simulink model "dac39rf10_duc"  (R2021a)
settings: Solver=FixedStepDiscrete  StartTime=0.0  StopTime=4136  RelTol=1e-3
StopFcn:
  | % Get interpolation factor from the L parameter on the DUC subsystem
  | duc = [gcs '/DUC']
  | Lstr = get_param(duc, 'L');
  | L = str2double(erase(Lstr, 'x'));
  | 
  | % Toss out 40*L output samples (40 input sample periods) for startup
  | N_in = size(dac_out,1)/L -40;
  | % Then assume input is bin-centered to the largest power of 2
  | N_in = 2^floor(log2(N_in));
  | % Multiply by L
  | N = N_in*L;
  | 
  | 
  | % Plot 2 channels
  | for ch = 0:1
  | 
  | 
  |     figure(ch+1);
  |     dac = dac_out(:,ch+1);
  |     dac_end = dac(end-N+1:end);
  |     f = [0:N/2];
  | 
  |     dac_fft = fft(dac_end/N*2);
  |     dac_fft = db( dac_fft(1:N/2+1) );
  |     dac_fft = max(dac_fft, -200*ones(N/2+1,1));
  | 
  |     plot(f, dac_fft);
  |     ylim([-150 3]);
  |     yticks([-200:10:0]);
  |     xlim([0 0.5]*N);
  |     xticks([0:0.5/8:0.5]*N);
  |     grid on;
  |     title(['DAC' num2str(ch) ' Output (' num2str(N) ' points)']);
  |     xlabel('Frequency Bin');
  |     ylabel('dBFS');
  | 
  | end
undefined symbols (not defined in the file): j, timearray
libraries: dspmlti4 x64, simulink x5
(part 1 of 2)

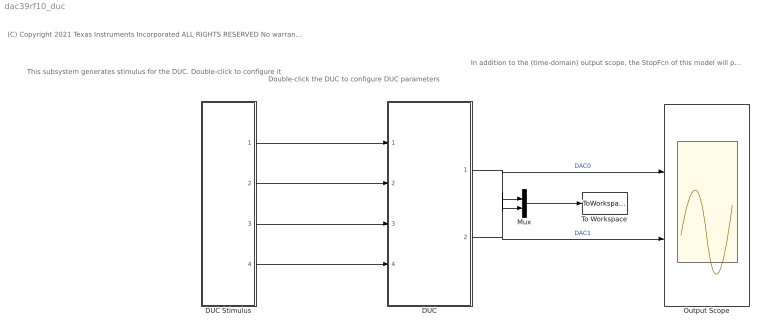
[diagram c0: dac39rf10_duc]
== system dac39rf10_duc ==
  note: Double-click the DUC to configure DUC parameters
  note: This subsystem generates stimulus for the DUC. Double-click to configure it
  note: In addition to the (time-domain) output scope, the StopFcn of this model will plot an FFT of the output
  note: (C) Copyright 2021 Texas Instruments Incorporated ALL RIGHTS RESERVED No warranty is expressed or implied
  DUC : Subsystem  mask{L=8x, DUC_FORMAT=off, FREQ0=0.25, FREQ1=0.25, FREQ2=0, FREQ3=0, PHASE0=0, PHASE1=0, PHASE2=0, PHASE3=0, DUC_GAIN0=-6dB, DUC_GAIN1=-6dB, DUC_GAIN2=0dB, DUC_GAIN3=0dB, DAC_SRC0_0=on, DAC_SRC0_1=on, DAC_SRC0_2=off, DAC_SRC0_3=off, DAC_SRC1_0=off, DAC_SRC1_1=on, DAC_SRC1_2=off, DAC_SRC1_3=off}
      mask prompts: L "Interpolation Factor"; DUC_FORMAT "Complex DUC Output (DUC_FORMAT=1)"; FREQ0 "Frequency (Ch 0) = 2^64 *"; FREQ1 "Frequency (Ch 1) = 2^64 *"; FREQ2 "Frequency (Ch 2) = 2^64 *"; FREQ3 "Frequency (Ch 3) = 2^64 *"; PHASE0 "Phase (Ch 0) = 2^16 *"; PHASE1 "Phase (Ch 1) = 2^16 *"; PHASE2 "Phase (Ch 2) = 2^16 *"; PHASE3 "Phase (Ch 3) = 2^16 *"; DAC_SRC0_0 "DUC0"; DAC_SRC0_1 "DUC1"; DAC_SRC0_2 "DUC2(real) / DUC0(imag)"; DAC_SRC0_3 "DUC3(real) / DUC1(imag)"; DAC_SRC1_0 "DUC0"; DAC_SRC1_1 "DUC1"; DAC_SRC1_2 "DUC2(real) / DUC0(imag)"; DAC_SRC1_3 "DUC3(real) / DUC1(imag)"
      mask help: DUC Model (DAC39RF10)
      mask init:
      | Lstr = get_param(gcb, 'L');
      | 
      | % Combine 4 frequency parameters into an array for the model to use
      | FREQ = [FREQ0 FREQ1 FREQ2 FREQ3];
      | 
      | PA_INIT = [PHASE0 PHASE1 PHASE2 PHASE3];
      | 
      | % Combine DAC_GAIN parameters
      | DUC_GAIN = [DUC_GAIN0 DUC_GAIN1 DUC_GAIN2 DUC_GAIN3];
      | 
      | % Convert 1->1, 2->0.5, 3->0.35
      | duc_gain = 2.^(1-DUC_GAIN);
      | 
      | % Combine DAC_SRC parameters into array for model
      | dac_src0 = [DAC_SRC0_0 DAC_SRC0_1 DAC_SRC0_2 DAC_SRC0_3];
      | dac_src1 = [DAC_SRC1_0 DAC_SRC1_1 DAC_SRC1_2 DAC_SRC1_3];
  DUC Stimulus : Subsystem  mask(Stimulus Block for DUC){N=4096, A0=0.99, F0=0.4, userData0=timearray, A1=0.99, F1=-0.4, userData1=, A2=0.99, F2=137/512, userData2=, A3=0.99, F3=137/512, userData3=}
      mask prompts: N "Sequence Length (N)"; A0 "Amplitude"; F0 "Frequency"; userData0 "User Data:"; A1 "Amplitude"; F1 "Frequency"; userData1 "User Data:"; A2 "Amplitude"; F2 "Frequency"; userData2 "User Data:"; A3 "Amplitude"; F3 "Frequency"; userData3 "User Data:"
      mask help: Specify Amplitudes and Frequencies for four IQ input channels. Sequency Length (N) should be a power of 2. The simulation stop time will be set to N+40 Amplitudes should be between 0.0 and 1.0 Frequencies units are [cycles per sample] (e.g. 1.0 = 2pi radians per sample) Frequencies outside the range of -0.5 to +0.5 will alias into that range. Frequencies will be rounded to make them coherent in N samples (length of input sequence) To provide custom stimulus, enter a variable name or MATLAB expression into the 'User Data' field. It will be evaluated in the base workspace, and should be a row or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
      mask init:
      | set_param(gcs, 'StopTime', num2str(N+40));
      | 
      | 
      | if( size(userData0,1) )
      |   duc0_input = evalin('base', userData0);
      | else
      |   duc0_input = A0*exp(j*round(F0*N)/N*2*pi*[0:N-1]) + (rand(1,N)-0.5)*2^-15;    
      | end
      | 
      | if( size(userData1,1) )
      |   duc1_input = evalin('base', userData1);
      | else
      |   duc1_input = A1*exp(j*round(F1*N)/N*2*pi*[0:N-1]) + (rand(1,N)-0.5)*2^-15;    
      | end
      | 
      | if( size(userData2,1) )
      |   duc2_input = evalin('base', userData2);
      | else
      |   duc2_input = A2*exp(j*round(F2*N)/N*2*pi*[0:N-1]) + (rand(1,N)-0.5)*2^-15;    
      | end
      | 
      | if( size(userData3,1) )
      |   duc3_input = evalin('base', userData3);
      | else
      |   duc3_input = A3*exp(j*round(F3*N)/N*2*pi*[0:N-1]) + (rand(1,N)-0.5)*2^-15;    
      | end
  Mux : Mux  Inputs=2
  Output Scope : Scope  NumInputPorts=2
  To Workspace : ToWorkspace  VariableName=dac_out  SampleTime=-1
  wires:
  DUC/1(Out1) -> Mux/1, Output Scope/1  "DAC0"
  DUC/2(Out2) -> Mux/2, Output Scope/2  "DAC1"
  Mux/1 -> To Workspace/1
  DUC Stimulus/1(Ch0) -> DUC/1(Ch0)
  DUC Stimulus/2(Ch1) -> DUC/2(Ch1)
  DUC Stimulus/3(Ch2) -> DUC/3(Ch2)
  DUC Stimulus/4(Ch3) -> DUC/4(Ch3)

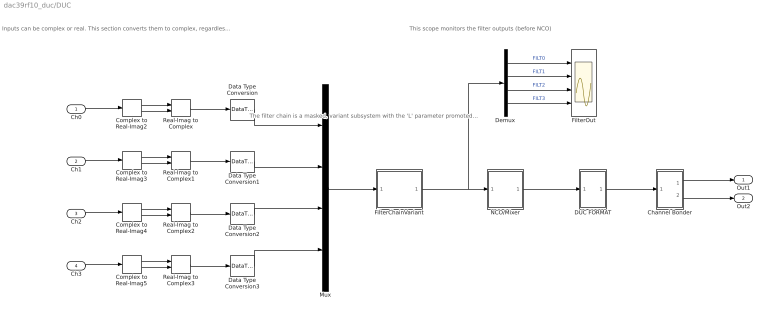
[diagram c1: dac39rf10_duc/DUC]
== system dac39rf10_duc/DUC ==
  note: This scope monitors the filter outputs (before NCO)
  note: The filter chain is a masked, variant subsystem with the 'L' parameter promoted up to the DUC mask
  note: Inputs can be complex or real. This section converts them to complex, regardless of what format they are initially in.
  Ch0 : Inport
  Ch1 : Inport  Port=2
  Ch2 : Inport  Port=3
  Ch3 : Inport  Port=4
  Channel Bonder : Subsystem
  Complex to Real-Imag{2..5} (4 alike) : ComplexToRealImag
  DUC FORMAT : Subsystem
  Data Type Conversion{,1..3} (4 alike) : DataTypeConversion  OutDataTypeStr=fixdt(1,16,15)  RndMeth=Round
  Demux : Demux
  FilterChainVariant : Subsystem  Variant=on  VariantControlMode=label  VariantControl=Variant1  LabelModeActiveChoice=var8x  mask{L=8x}
      mask prompts: L "Interpolation Factor"
      mask init:
      | simulationStatus =  get_param(bdroot,'SimulationStatus');
      | 
      | % The active variant can only be modified at edit-time or very early during
      | % the simulink compile stage. 
      | 
      |    % The L parameter is just an index into a list of strings. This gets the
      |    % string
      |    Lstr = get_param(gcb, 'L');  
      |    set_param(gcb, 'OverrideUsingVariant', ['var', Lstr]);
  FilterOut : Scope  NumInputPorts=4
  Mux : Mux
  NCO/Mixer : Subsystem
  Real-Imag to Complex{,1..3} (4 alike) : RealImagToComplex
  Out1 : Outport  VectorParamsAs1DForOutWhenUnconnected=off
  Out2 : Outport  Port=2  VectorParamsAs1DForOutWhenUnconnected=off
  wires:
  Demux/2 -> FilterOut/2  "FILT1"
  Demux/1 -> FilterOut/1  "FILT0"
  Mux/1 -> FilterChainVariant/1("In1 ")
  Complex to Real-Imag2/1 -> Real-Imag to Complex/1
  Complex to Real-Imag2/2 -> Real-Imag to Complex/2
  Complex to Real-Imag3/2 -> Real-Imag to Complex1/2
  Complex to Real-Imag3/1 -> Real-Imag to Complex1/1
  Complex to Real-Imag4/1 -> Real-Imag to Complex2/1
  Complex to Real-Imag4/2 -> Real-Imag to Complex2/2
  Complex to Real-Imag5/2 -> Real-Imag to Complex3/2
  Complex to Real-Imag5/1 -> Real-Imag to Complex3/1
  Ch0/1 -> Complex to Real-Imag2/1
  Ch1/1 -> Complex to Real-Imag3/1
  Ch2/1 -> Complex to Real-Imag4/1
  Ch3/1 -> Complex to Real-Imag5/1
  Real-Imag to Complex/1 -> Data Type Conversion/1
  Real-Imag to Complex1/1 -> Data Type Conversion1/1
  Real-Imag to Complex2/1 -> Data Type Conversion2/1
  Real-Imag to Complex3/1 -> Data Type Conversion3/1
  FilterChainVariant/1(" Out1") -> Demux/1, NCO/Mixer/1(In1)
  NCO/Mixer/1(Out1) -> DUC FORMAT/1(In1)
  DUC FORMAT/1(Out1) -> Channel Bonder/1(In1)
  Channel Bonder/1(Out1) -> Out1/1
  Channel Bonder/2(Out2) -> Out2/1
  Demux/3 -> FilterOut/3  "FILT2"
  Demux/4 -> FilterOut/4  "FILT3"
  Data Type Conversion/1 -> Mux/1
  Data Type Conversion1/1 -> Mux/2
  Data Type Conversion2/1 -> Mux/3
  Data Type Conversion3/1 -> Mux/4

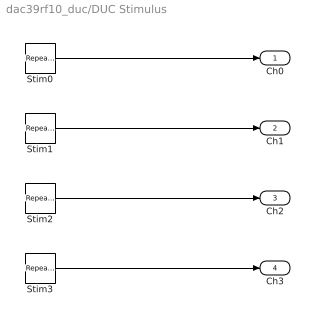
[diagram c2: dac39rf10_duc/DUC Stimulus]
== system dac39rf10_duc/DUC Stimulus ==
  Stim0 : simulink/Sources/Repeating Sequence Stair  OutValues=duc0_input  tsamp=1  OutMin=[]  OutMax=[]  OutDataTypeStr=double  OutputDataTypeScalingMode=double  OutDataType=fixdt(0,8)  ConRadixGroup=Best Precision: Vector-wise  OutScaling=2^-12
  Stim1 : simulink/Sources/Repeating Sequence Stair  OutValues=duc1_input  tsamp=1  OutMin=[]  OutMax=[]  OutDataTypeStr=double  OutputDataTypeScalingMode=double  OutDataType=fixdt(0,8)  ConRadixGroup=Best Precision: Vector-wise  OutScaling=2^-12
  Stim2 : simulink/Sources/Repeating Sequence Stair  OutValues=duc2_input  tsamp=1  OutMin=[]  OutMax=[]  OutDataTypeStr=double  OutputDataTypeScalingMode=double  OutDataType=fixdt(0,8)  ConRadixGroup=Best Precision: Vector-wise  OutScaling=2^-12
  Stim3 : simulink/Sources/Repeating Sequence Stair  OutValues=duc3_input  tsamp=1  OutMin=[]  OutMax=[]  OutDataTypeStr=double  OutputDataTypeScalingMode=double  OutDataType=fixdt(0,8)  ConRadixGroup=Best Precision: Vector-wise  OutScaling=2^-12
  Ch0 : Outport  VectorParamsAs1DForOutWhenUnconnected=off
  Ch1 : Outport  Port=2  VectorParamsAs1DForOutWhenUnconnected=off
  Ch2 : Outport  Port=3  VectorParamsAs1DForOutWhenUnconnected=off
  Ch3 : Outport  Port=4  VectorParamsAs1DForOutWhenUnconnected=off
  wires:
  Stim1/1 -> Ch1/1
  Stim2/1 -> Ch2/1
  Stim3/1 -> Ch3/1
  Stim0/1 -> Ch0/1

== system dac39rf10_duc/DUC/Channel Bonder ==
  note: DUC_GAIN is done with elementwise multiplication
  note: DAC_SRC is done with matrix multiplication (1x4 * 4x1 = 1x1)
  In1 : Inport  PortDimensions=4
  DAC_SRC0 : Gain  Gain=dac_src0  Multiplication=Matrix(K*u)  OutDataTypeStr=fixdt(1,16,15)  RndMeth=Nearest
  DAC_SRC1 : Gain  Gain=dac_src1  Multiplication=Matrix(K*u)  OutDataTypeStr=fixdt(1,16,15)  RndMeth=Nearest
  DUC_GAIN : Gain  Gain=duc_gain  OutDataTypeStr=fixdt(1,18,17)
  Out1 : Outport  VectorParamsAs1DForOutWhenUnconnected=off
  Out2 : Outport  Port=2  VectorParamsAs1DForOutWhenUnconnected=off
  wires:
  DAC_SRC0/1 -> Out1/1
  DUC_GAIN/1 -> DAC_SRC1/1, DAC_SRC0/1
  DAC_SRC1/1 -> Out2/1
  In1/1 -> DUC_GAIN/1

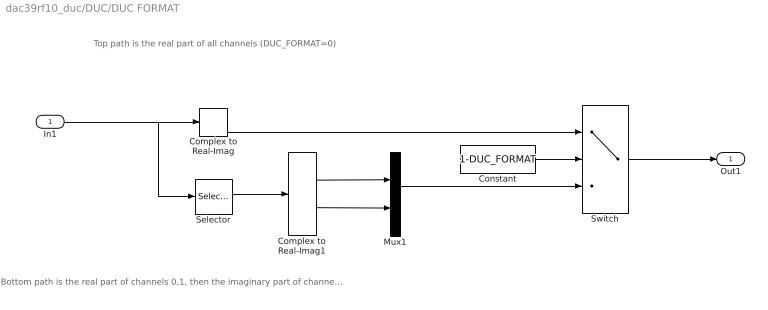
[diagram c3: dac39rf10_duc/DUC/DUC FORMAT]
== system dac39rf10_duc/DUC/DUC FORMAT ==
  note: Bottom path is the real part of channels 0,1, then the imaginary part of channels 0 and 1 (DUC_FORMAT=1)
  note: Top path is the real part of all channels (DUC_FORMAT=0)
  In1 : Inport  PortDimensions=4
  Complex to Real-Imag : ComplexToRealImag  Output=Real
  Complex to Real-Imag1 : ComplexToRealImag
  Constant : Constant  Value=1-DUC_FORMAT
  Mux1 : Mux  Inputs=2
  Selector : Selector  InputPortWidth=4  IndexOptions=Index vector (dialog)  Indices=[1 2]  OutputSizes=1
  Switch : Switch  Criteria=u2 > Threshold
  Out1 : Outport  PortDimensions=4  VectorParamsAs1DForOutWhenUnconnected=off
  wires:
  Mux1/1 -> Switch/3
  Complex to Real-Imag/1 -> Switch/1
  Complex to Real-Imag1/1 -> Mux1/1
  Selector/1 -> Complex to Real-Imag1/1
  In1/1 -> Selector/1, Complex to Real-Imag/1
  Switch/1 -> Out1/1
  Complex to Real-Imag1/2 -> Mux1/2
  Constant/1 -> Switch/2

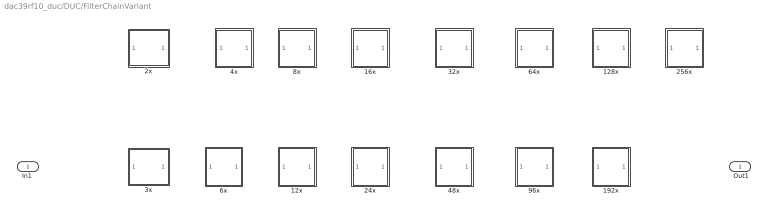
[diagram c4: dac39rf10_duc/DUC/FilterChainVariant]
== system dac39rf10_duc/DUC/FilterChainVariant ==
  "In1 " : Inport
  128x : Subsystem  VariantControl=var128x
  12x : Subsystem  VariantControl=var12x
  16x : Subsystem  VariantControl=var16x
  192x : Subsystem  VariantControl=var192x
  24x : Subsystem  VariantControl=var24x
  256x : Subsystem  VariantControl=var256x
  2x : Subsystem  VariantControl=var2x
  32x : Subsystem  VariantControl=var32x
  3x : Subsystem  VariantControl=var3x
  48x : Subsystem  VariantControl=var48x
  4x : Subsystem  VariantControl=var4x
  64x : Subsystem  VariantControl=var64x
  6x : Subsystem  VariantControl=var6x
  8x : Subsystem  VariantControl=var8x
  96x : Subsystem  VariantControl=var96x
  " Out1" : Outport  VectorParamsAs1DForOutWhenUnconnected=off

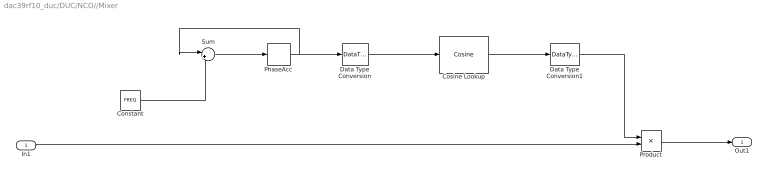
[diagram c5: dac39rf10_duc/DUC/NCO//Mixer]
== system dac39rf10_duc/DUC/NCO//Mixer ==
  In1 : Inport
  Constant : Constant  Value=FREQ  OutDataTypeStr=fixdt(0,64,64)
  Cosine Lookup : simulink/Lookup Tables/Cosine  Formula=exp(j*2*pi*u)  NumDataPoints=(2^18)+1  OutputWordLength=20  InternalRulePriority=Precision
  Data Type Conversion : DataTypeConversion  OutDataTypeStr=fixdt(0,18,18)
  Data Type Conversion1 : DataTypeConversion  OutDataTypeStr=fixdt(1,17,15)  RndMeth=Nearest
  PhaseAcc : Delay  DelayLength=1  InitialCondition=PA_INIT
  Product : Product  OutDataTypeStr=fixdt(1,16,15)  RndMeth=Nearest  SaturateOnIntegerOverflow=on
  Sum : Sum  Inputs=|++  OutDataTypeStr=fixdt(0,64,64)
  Out1 : Outport  VectorParamsAs1DForOutWhenUnconnected=off
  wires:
  PhaseAcc/1 -> Sum/1, Data Type Conversion/1
  Product/1 -> Out1/1
  In1/1 -> Product/2
  Cosine Lookup/1 -> Data Type Conversion1/1
  Data Type Conversion1/1 -> Product/1
  Sum/1 -> PhaseAcc/1
  Data Type Conversion/1 -> Cosine Lookup/1
  Constant/1 -> Sum/2

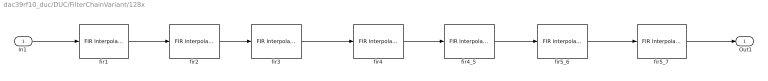
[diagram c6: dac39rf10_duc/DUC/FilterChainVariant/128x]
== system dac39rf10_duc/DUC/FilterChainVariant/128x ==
  "In1 " : Inport
  fir1 : dspmlti4/FIR Interpolation  FilterSource=Dialog parameters  h=[6 0 -19 0 47 0 -100 0 192 0 -342 0 572 0 -914 0 1409 0 -2119 0 3152 0 -4729 0 7420 0 -13334 0 41527 65536 41527 0 -13334 0 7420 0 -4729 0 3152 0 -2119 0 1409 0 -914 0 572 0 -342 0 192 0 -100 0 47 0 -19 0 6 ]*2^-16  L=2  FilterObject=FINTERP  framing=Enforce single-rate processing  outputBufInitCond=0  roundingMode=Round  overflowMode=on  firstCoeffMode=Binary point scaling  firstCoeffWordLength=18  firstCoeffFracLength=16  firstCoeffDataTypeStr=fixdt(1,18,16)  firstCoeffMin=[]  firstCoeffMax=[]  firstCoeffLastDataTypeStr=fixdt(1,18,16)  outputMode=Binary point scaling  outputWordLength=18  outputFracLength=17  outputDataTypeStr=fixdt(1,18,17)  outputMin=[]  outputMax=[]  outputLastDataTypeStr=fixdt(1,18,17)
  fir2 : dspmlti4/FIR Interpolation  FilterSource=Dialog parameters  h=[-12 0 84 0 -336 0 1006 0 -2691 0 10141 16384 10141 0 -2691 0 1006 0 -336 0 84 0 -12 ]*2^-14  L=2  FilterObject=FINTERP  framing=Enforce single-rate processing  outputBufInitCond=0  roundingMode=Round  overflowMode=on  firstCoeffMode=Binary point scaling  firstCoeffWordLength=16  firstCoeffFracLength=14  firstCoeffDataTypeStr=fixdt(1,16,14)  firstCoeffMin=[]  firstCoeffMax=[]  firstCoeffLastDataTypeStr=fixdt(1,16,14)  outputMode=Binary point scaling  outputWordLength=18  outputFracLength=17  outputDataTypeStr=fixdt(1,18,17)  outputMin=[]  outputMax=[]  outputLastDataTypeStr=fixdt(1,18,17)
  fir3 : dspmlti4/FIR Interpolation  FilterSource=Dialog parameters  h=[29 0 -214 0 1209 2048 1209 0 -214 0 29 ]*2^-11  L=2  FilterObject=FINTERP  framing=Enforce single-rate processing  outputBufInitCond=0  roundingMode=Round  overflowMode=on  firstCoeffMode=Binary point scaling  firstCoeffWordLength=13  firstCoeffFracLength=11  firstCoeffDataTypeStr=fixdt(1,13,11)  firstCoeffMin=[]  firstCoeffMax=[]  firstCoeffLastDataTypeStr=fixdt(1,13,11)  outputMode=Binary point scaling  outputWordLength=17  outputFracLength=16  outputDataTypeStr=fixdt(1,17,16)  outputMin=[]  outputMax=[]  outputLastDataTypeStr=fixdt(1,17,16)
  fir4 : dspmlti4/FIR Interpolation  FilterSource=Dialog parameters  h=[3 0 -25 0 150 256 150 0 -25 0 3 ]*2^-8  L=2  FilterObject=FINTERP  framing=Enforce single-rate processing  outputBufInitCond=0  roundingMode=Round  overflowMode=on  firstCoeffMode=Binary point scaling  firstCoeffWordLength=10  firstCoeffFracLength=8  firstCoeffDataTypeStr=fixdt(1,10,8)  firstCoeffMin=[]  firstCoeffMax=[]  firstCoeffLastDataTypeStr=fixdt(1,10,8)  outputMode=Binary point scaling  outputWordLength=17  outputFracLength=16  outputDataTypeStr=fixdt(1,17,16)  outputMin=[]  outputMax=[]  outputLastDataTypeStr=fixdt(1,17,16)
  fir4_5 : dspmlti4/FIR Interpolation  FilterSource=Dialog parameters  h=[3 0 -25 0 150 256 150 0 -25 0 3 ]*2^-8  L=2  FilterObject=FINTERP  framing=Enforce single-rate processing  outputBufInitCond=0  roundingMode=Round  overflowMode=on  firstCoeffMode=Binary point scaling  firstCoeffWordLength=10  firstCoeffFracLength=8  firstCoeffDataTypeStr=fixdt(1,10,8)  firstCoeffMin=[]  firstCoeffMax=[]  firstCoeffLastDataTypeStr=fixdt(1,10,8)  outputMode=Binary point scaling  outputWordLength=17  outputFracLength=16  outputDataTypeStr=fixdt(1,17,16)  outputMin=[]  outputMax=[]  outputLastDataTypeStr=fixdt(1,17,16)
  fir5_6 : dspmlti4/FIR Interpolation  FilterSource=Dialog parameters  h=[-1 0 9 16 9 0 -1]*2^-4  L=2  FilterObject=FINTERP  framing=Enforce single-rate processing  outputBufInitCond=0  roundingMode=Round  overflowMode=on  firstCoeffMode=Binary point scaling  firstCoeffWordLength=6  firstCoeffFracLength=4  firstCoeffDataTypeStr=fixdt(1,6,4)  firstCoeffMin=[]  firstCoeffMax=[]  firstCoeffLastDataTypeStr=fixdt(1,6,4)  outputMode=Binary point scaling  outputWordLength=16  outputFracLength=15  outputDataTypeStr=fixdt(1,16,15)  outputMin=[]  outputMax=[]  outputLastDataTypeStr=fixdt(1,16,15)
  fir5_7 : dspmlti4/FIR Interpolation  FilterSource=Dialog parameters  h=[-1 0 9 16 9 0 -1]*2^-4  L=2  FilterObject=FINTERP  framing=Enforce single-rate processing  outputBufInitCond=0  roundingMode=Round  overflowMode=on  firstCoeffMode=Binary point scaling  firstCoeffWordLength=6  firstCoeffFracLength=4  firstCoeffDataTypeStr=fixdt(1,6,4)  firstCoeffMin=[]  firstCoeffMax=[]  firstCoeffLastDataTypeStr=fixdt(1,6,4)  outputMode=Binary point scaling  outputWordLength=16  outputFracLength=15  outputDataTypeStr=fixdt(1,16,15)  outputMin=[]  outputMax=[]  outputLastDataTypeStr=fixdt(1,16,15)
  " Out1" : Outport  VectorParamsAs1DForOutWhenUnconnected=off
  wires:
  fir5_7/1 -> " Out1"/1
  fir4/1 -> fir4_5/1
  fir3/1 -> fir4/1
  fir2/1 -> fir3/1
  fir1/1 -> fir2/1
  "In1 "/1 -> fir1/1
  fir5_6/1 -> fir5_7/1
  fir4_5/1 -> fir5_6/1

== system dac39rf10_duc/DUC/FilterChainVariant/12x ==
  "In1 " : Inport
  fir2 : dspmlti4/FIR Interpolation  FilterSource=Dialog parameters  h=[-12 0 84 0 -336 0 1006 0 -2691 0 10141 16384 10141 0 -2691 0 1006 0 -336 0 84 0 -12 ]*2^-14  L=2  FilterObject=FINTERP  framing=Enforce single-rate processing  outputBufInitCond=0  roundingMode=Round  overflowMode=on  firstCoeffMode=Binary point scaling  firstCoeffWordLength=16  firstCoeffFracLength=14  firstCoeffDataTypeStr=fixdt(1,16,14)  firstCoeffMin=[]  firstCoeffMax=[]  firstCoeffLastDataTypeStr=fixdt(1,16,14)  outputMode=Binary point scaling  outputWordLength=18  outputFracLength=17  outputDataTypeStr=fixdt(1,18,17)  outputMin=[]  outputMax=[]  outputLastDataTypeStr=fixdt(1,18,17)
  fir3 : dspmlti4/FIR Interpolation  FilterSource=Dialog parameters  h=[29 0 -214 0 1209 2048 1209 0 -214 0 29 ]*2^-11  L=2  FilterObject=FINTERP  framing=Enforce single-rate processing  outputBufInitCond=0  roundingMode=Round  overflowMode=on  firstCoeffMode=Binary point scaling  firstCoeffWordLength=13  firstCoeffFracLength=11  firstCoeffDataTypeStr=fixdt(1,13,11)  firstCoeffMin=[]  firstCoeffMax=[]  firstCoeffLastDataTypeStr=fixdt(1,13,11)  outputMode=Binary point scaling  outputWordLength=16  outputFracLength=15  outputDataTypeStr=fixdt(1,16,15)  outputMin=[]  outputMax=[]  outputLastDataTypeStr=fixdt(1,16,15)
  fir3x : dspmlti4/FIR Interpolation  FilterSource=Dialog parameters  h=[-38 -38 0 83 117 0 -214 -281 0 464 584 0 -900 -1102 0 1612 1929 0 -2713 -3190 0 4346 5040 0 -6699 -7684 0 10023 11408 0 -14701 -16661 0 21389 24260 0 -31417 -35960 0 48101 56540 0 -82781 -105224 0 215190 432780 524288 432780 215190 0 -105224 -82781 0 56540 48101 0 -35960 -31417 0 24260 21389 0 -16661 -14701 0 11408 10023 0 -7684 -6699 0 5040 4346 0 -3190 -2713 0 1929 1612 0 -1102 -900 0 584 464 0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  L=3  FilterObject=FINTERP  framing=Enforce single-rate processing  outputBufInitCond=0  roundingMode=Round  overflowMode=on  firstCoeffMode=Binary point scaling  firstCoeffWordLength=21  firstCoeffFracLength=19  firstCoeffDataTypeStr=fixdt(1,21,19)  firstCoeffMin=[]  firstCoeffMax=[]  firstCoeffLastDataTypeStr=fixdt(1,21,19)  outputMode=Binary point scaling  outputWordLength=18  outputFracLength=17  outputDataTypeStr=fixdt(1,18,17)  outputMin=[]  outputMax=[]  outputLastDataTypeStr=fixdt(1,18,17)
  " Out1" : Outport  VectorParamsAs1DForOutWhenUnconnected=off
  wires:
  fir3/1 -> " Out1"/1
  "In1 "/1 -> fir3x/1
  fir3x/1 -> fir2/1
  fir2/1 -> fir3/1

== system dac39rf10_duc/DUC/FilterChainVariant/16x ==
  "In1 " : Inport
  fir1 : dspmlti4/FIR Interpolation  FilterSource=Dialog parameters  h=[6 0 -19 0 47 0 -100 0 192 0 -342 0 572 0 -914 0 1409 0 -2119 0 3152 0 -4729 0 7420 0 -13334 0 41527 65536 41527 0 -13334 0 7420 0 -4729 0 3152 0 -2119 0 1409 0 -914 0 572 0 -342 0 192 0 -100 0 47 0 -19 0 6 ]*2^-16  L=2  FilterObject=FINTERP  framing=Enforce single-rate processing  outputBufInitCond=0  roundingMode=Round  overflowMode=on  firstCoeffMode=Binary point scaling  firstCoeffWordLength=18  firstCoeffFracLength=16  firstCoeffDataTypeStr=fixdt(1,18,16)  firstCoeffMin=[]  firstCoeffMax=[]  firstCoeffLastDataTypeStr=fixdt(1,18,16)  outputMode=Binary point scaling  outputWordLength=18  outputFracLength=17  outputDataTypeStr=fixdt(1,18,17)  outputMin=[]  outputMax=[]  outputLastDataTypeStr=fixdt(1,18,17)
  fir2 : dspmlti4/FIR Interpolation  FilterSource=Dialog parameters  h=[-12 0 84 0 -336 0 1006 0 -2691 0 10141 16384 10141 0 -2691 0 1006 0 -336 0 84 0 -12 ]*2^-14  L=2  FilterObject=FINTERP  framing=Enforce single-rate processing  outputBufInitCond=0  roundingMode=Round  overflowMode=on  firstCoeffMode=Binary point scaling  firstCoeffWordLength=16  firstCoeffFracLength=14  firstCoeffDataTypeStr=fixdt(1,16,14)  firstCoeffMin=[]  firstCoeffMax=[]  firstCoeffLastDataTypeStr=fixdt(1,16,14)  outputMode=Binary point scaling  outputWordLength=18  outputFracLength=17  outputDataTypeStr=fixdt(1,18,17)  outputMin=[]  outputMax=[]  outputLastDataTypeStr=fixdt(1,18,17)
  fir3 : dspmlti4/FIR Interpolation  FilterSource=Dialog parameters  h=[29 0 -214 0 1209 2048 1209 0 -214 0 29 ]*2^-11  L=2  FilterObject=FINTERP  framing=Enforce single-rate processing  outputBufInitCond=0  roundingMode=Round  overflowMode=on  firstCoeffMode=Binary point scaling  firstCoeffWordLength=13  firstCoeffFracLength=11  firstCoeffDataTypeStr=fixdt(1,13,11)  firstCoeffMin=[]  firstCoeffMax=[]  firstCoeffLastDataTypeStr=fixdt(1,13,11)  outputMode=Binary point scaling  outputWordLength=17  outputFracLength=16  outputDataTypeStr=fixdt(1,17,16)  outputMin=[]  outputMax=[]  outputLastDataTypeStr=fixdt(1,17,16)
  fir4 : dspmlti4/FIR Interpolation  FilterSource=Dialog parameters  h=[3 0 -25 0 150 256 150 0 -25 0 3 ]*2^-8  L=2  FilterObject=FINTERP  framing=Enforce single-rate processing  outputBufInitCond=0  roundingMode=Round  overflowMode=on  firstCoeffMode=Binary point scaling  firstCoeffWordLength=10  firstCoeffFracLength=8  firstCoeffDataTypeStr=fixdt(1,10,8)  firstCoeffMin=[]  firstCoeffMax=[]  firstCoeffLastDataTypeStr=fixdt(1,10,8)  outputMode=Binary point scaling  outputWordLength=16  outputFracLength=15  outputDataTypeStr=fixdt(1,16,15)  outputMin=[]  outputMax=[]  outputLastDataTypeStr=fixdt(1,16,15)
  " Out1" : Outport  VectorParamsAs1DForOutWhenUnconnected=off
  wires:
  "In1 "/1 -> fir1/1
  fir1/1 -> fir2/1
  fir2/1 -> fir3/1
  fir3/1 -> fir4/1
  fir4/1 -> " Out1"/1

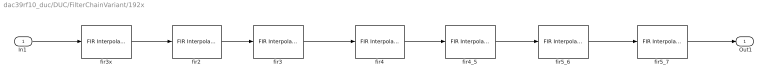
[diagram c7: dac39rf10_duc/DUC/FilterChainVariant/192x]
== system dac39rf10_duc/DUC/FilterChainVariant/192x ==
  "In1 " : Inport
  fir2 : dspmlti4/FIR Interpolation  FilterSource=Dialog parameters  h=[-12 0 84 0 -336 0 1006 0 -2691 0 10141 16384 10141 0 -2691 0 1006 0 -336 0 84 0 -12 ]*2^-14  L=2  FilterObject=FINTERP  framing=Enforce single-rate processing  outputBufInitCond=0  roundingMode=Round  overflowMode=on  firstCoeffMode=Binary point scaling  firstCoeffWordLength=16  firstCoeffFracLength=14  firstCoeffDataTypeStr=fixdt(1,16,14)  firstCoeffMin=[]  firstCoeffMax=[]  firstCoeffLastDataTypeStr=fixdt(1,16,14)  outputMode=Binary point scaling  outputWordLength=18  outputFracLength=17  outputDataTypeStr=fixdt(1,18,17)  outputMin=[]  outputMax=[]  outputLastDataTypeStr=fixdt(1,18,17)
  fir3 : dspmlti4/FIR Interpolation  FilterSource=Dialog parameters  h=[29 0 -214 0 1209 2048 1209 0 -214 0 29 ]*2^-11  L=2  FilterObject=FINTERP  framing=Enforce single-rate processing  outputBufInitCond=0  roundingMode=Round  overflowMode=on  firstCoeffMode=Binary point scaling  firstCoeffWordLength=13  firstCoeffFracLength=11  firstCoeffDataTypeStr=fixdt(1,13,11)  firstCoeffMin=[]  firstCoeffMax=[]  firstCoeffLastDataTypeStr=fixdt(1,13,11)  outputMode=Binary point scaling  outputWordLength=17  outputFracLength=16  outputDataTypeStr=fixdt(1,17,16)  outputMin=[]  outputMax=[]  outputLastDataTypeStr=fixdt(1,17,16)
  fir3x : dspmlti4/FIR Interpolation  FilterSource=Dialog parameters  h=[-38 -38 0 83 117 0 -214 -281 0 464 584 0 -900 -1102 0 1612 1929 0 -2713 -3190 0 4346 5040 0 -6699 -7684 0 10023 11408 0 -14701 -16661 0 21389 24260 0 -31417 -35960 0 48101 56540 0 -82781 -105224 0 215190 432780 524288 432780 215190 0 -105224 -82781 0 56540 48101 0 -35960 -31417 0 24260 21389 0 -16661 -14701 0 11408 10023 0 -7684 -6699 0 5040 4346 0 -3190 -2713 0 1929 1612 0 -1102 -900 0 584 464 0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  L=3  FilterObject=FINTERP  framing=Enforce single-rate processing  outputBufInitCond=0  roundingMode=Round  overflowMode=on  firstCoeffMode=Binary point scaling  firstCoeffWordLength=21  firstCoeffFracLength=19  firstCoeffDataTypeStr=fixdt(1,21,19)  firstCoeffMin=[]  firstCoeffMax=[]  firstCoeffLastDataTypeStr=fixdt(1,21,19)  outputMode=Binary point scaling  outputWordLength=18  outputFracLength=17  outputDataTypeStr=fixdt(1,18,17)  outputMin=[]  outputMax=[]  outputLastDataTypeStr=fixdt(1,18,17)
  fir4 : dspmlti4/FIR Interpolation  FilterSource=Dialog parameters  h=[3 0 -25 0 150 256 150 0 -25 0 3 ]*2^-8  L=2  FilterObject=FINTERP  framing=Enforce single-rate processing  outputBufInitCond=0  roundingMode=Round  overflowMode=on  firstCoeffMode=Binary point scaling  firstCoeffWordLength=10  firstCoeffFracLength=8  firstCoeffDataTypeStr=fixdt(1,10,8)  firstCoeffMin=[]  firstCoeffMax=[]  firstCoeffLastDataTypeStr=fixdt(1,10,8)  outputMode=Binary point scaling  outputWordLength=17  outputFracLength=16  outputDataTypeStr=fixdt(1,17,16)  outputMin=[]  outputMax=[]  outputLastDataTypeStr=fixdt(1,17,16)
  fir4_5 : dspmlti4/FIR Interpolation  FilterSource=Dialog parameters  h=[3 0 -25 0 150 256 150 0 -25 0 3 ]*2^-8  L=2  FilterObject=FINTERP  framing=Enforce single-rate processing  outputBufInitCond=0  roundingMode=Round  overflowMode=on  firstCoeffMode=Binary point scaling  firstCoeffWordLength=10  firstCoeffFracLength=8  firstCoeffDataTypeStr=fixdt(1,10,8)  firstCoeffMin=[]  firstCoeffMax=[]  firstCoeffLastDataTypeStr=fixdt(1,10,8)  outputMode=Binary point scaling  outputWordLength=17  outputFracLength=16  outputDataTypeStr=fixdt(1,17,16)  outputMin=[]  outputMax=[]  outputLastDataTypeStr=fixdt(1,17,16)
  fir5_6 : dspmlti4/FIR Interpolation  FilterSource=Dialog parameters  h=[-1 0 9 16 9 0 -1]*2^-4  L=2  FilterObject=FINTERP  framing=Enforce single-rate processing  outputBufInitCond=0  roundingMode=Round  overflowMode=on  firstCoeffMode=Binary point scaling  firstCoeffWordLength=6  firstCoeffFracLength=4  firstCoeffDataTypeStr=fixdt(1,6,4)  firstCoeffMin=[]  firstCoeffMax=[]  firstCoeffLastDataTypeStr=fixdt(1,6,4)  outputMode=Binary point scaling  outputWordLength=16  outputFracLength=15  outputDataTypeStr=fixdt(1,16,15)  outputMin=[]  outputMax=[]  outputLastDataTypeStr=fixdt(1,16,15)
  fir5_7 : dspmlti4/FIR Interpolation  FilterSource=Dialog parameters  h=[-1 0 9 16 9 0 -1]*2^-4  L=2  FilterObject=FINTERP  framing=Enforce single-rate processing  outputBufInitCond=0  roundingMode=Round  overflowMode=on  firstCoeffMode=Binary point scaling  firstCoeffWordLength=6  firstCoeffFracLength=4  firstCoeffDataTypeStr=fixdt(1,6,4)  firstCoeffMin=[]  firstCoeffMax=[]  firstCoeffLastDataTypeStr=fixdt(1,6,4)  outputMode=Binary point scaling  outputWordLength=16  outputFracLength=15  outputDataTypeStr=fixdt(1,16,15)  outputMin=[]  outputMax=[]  outputLastDataTypeStr=fixdt(1,16,15)
  " Out1" : Outport  VectorParamsAs1DForOutWhenUnconnected=off
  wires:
  fir4_5/1 -> fir5_6/1
  fir5_6/1 -> fir5_7/1
  "In1 "/1 -> fir3x/1
  fir3x/1 -> fir2/1
  fir2/1 -> fir3/1
  fir3/1 -> fir4/1
  fir4/1 -> fir4_5/1
  fir5_7/1 -> " Out1"/1

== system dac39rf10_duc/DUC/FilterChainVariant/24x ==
  "In1 " : Inport
  fir2 : dspmlti4/FIR Interpolation  FilterSource=Dialog parameters  h=[-12 0 84 0 -336 0 1006 0 -2691 0 10141 16384 10141 0 -2691 0 1006 0 -336 0 84 0 -12 ]*2^-14  L=2  FilterObject=FINTERP  framing=Enforce single-rate processing  outputBufInitCond=0  roundingMode=Round  overflowMode=on  firstCoeffMode=Binary point scaling  firstCoeffWordLength=16  firstCoeffFracLength=14  firstCoeffDataTypeStr=fixdt(1,16,14)  firstCoeffMin=[]  firstCoeffMax=[]  firstCoeffLastDataTypeStr=fixdt(1,16,14)  outputMode=Binary point scaling  outputWordLength=18  outputFracLength=17  outputDataTypeStr=fixdt(1,18,17)  outputMin=[]  outputMax=[]  outputLastDataTypeStr=fixdt(1,18,17)
  fir3 : dspmlti4/FIR Interpolation  FilterSource=Dialog parameters  h=[29 0 -214 0 1209 2048 1209 0 -214 0 29 ]*2^-11  L=2  FilterObject=FINTERP  framing=Enforce single-rate processing  outputBufInitCond=0  roundingMode=Round  overflowMode=on  firstCoeffMode=Binary point scaling  firstCoeffWordLength=13  firstCoeffFracLength=11  firstCoeffDataTypeStr=fixdt(1,13,11)  firstCoeffMin=[]  firstCoeffMax=[]  firstCoeffLastDataTypeStr=fixdt(1,13,11)  outputMode=Binary point scaling  outputWordLength=17  outputFracLength=16  outputDataTypeStr=fixdt(1,17,16)  outputMin=[]  outputMax=[]  outputLastDataTypeStr=fixdt(1,17,16)
  fir3x : dspmlti4/FIR Interpolation  FilterSource=Dialog parameters  h=[-38 -38 0 83 117 0 -214 -281 0 464 584 0 -900 -1102 0 1612 1929 0 -2713 -3190 0 4346 5040 0 -6699 -7684 0 10023 11408 0 -14701 -16661 0 21389 24260 0 -31417 -35960 0 48101 56540 0 -82781 -105224 0 215190 432780 524288 432780 215190 0 -105224 -82781 0 56540 48101 0 -35960 -31417 0 24260 21389 0 -16661 -14701 0 11408 10023 0 -7684 -6699 0 5040 4346 0 -3190 -2713 0 1929 1612 0 -1102 -900 0 584 464 0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  L=3  FilterObject=FINTERP  framing=Enforce single-rate processing  outputBufInitCond=0  roundingMode=Round  overflowMode=on  firstCoeffMode=Binary point scaling  firstCoeffWordLength=21  firstCoeffFracLength=19  firstCoeffDataTypeStr=fixdt(1,21,19)  firstCoeffMin=[]  firstCoeffMax=[]  firstCoeffLastDataTypeStr=fixdt(1,21,19)  outputMode=Binary point scaling  outputWordLength=18  outputFracLength=17  outputDataTypeStr=fixdt(1,18,17)  outputMin=[]  outputMax=[]  outputLastDataTypeStr=fixdt(1,18,17)
  fir4 : dspmlti4/FIR Interpolation  FilterSource=Dialog parameters  h=[3 0 -25 0 150 256 150 0 -25 0 3 ]*2^-8  L=2  FilterObject=FINTERP  framing=Enforce single-rate processing  outputBufInitCond=0  roundingMode=Round  overflowMode=on  firstCoeffMode=Binary point scaling  firstCoeffWordLength=10  firstCoeffFracLength=8  firstCoeffDataTypeStr=fixdt(1,10,8)  firstCoeffMin=[]  firstCoeffMax=[]  firstCoeffLastDataTypeStr=fixdt(1,10,8)  outputMode=Binary point scaling  outputWordLength=16  outputFracLength=15  outputDataTypeStr=fixdt(1,16,15)  outputMin=[]  outputMax=[]  outputLastDataTypeStr=fixdt(1,16,15)
  " Out1" : Outport  VectorParamsAs1DForOutWhenUnconnected=off
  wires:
  fir4/1 -> " Out1"/1
  fir3/1 -> fir4/1
  fir2/1 -> fir3/1
  fir3x/1 -> fir2/1
  "In1 "/1 -> fir3x/1

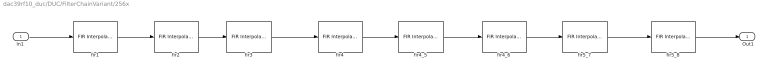
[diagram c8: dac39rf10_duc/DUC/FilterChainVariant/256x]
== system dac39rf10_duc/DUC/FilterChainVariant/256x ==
  "In1 " : Inport
  fir1 : dspmlti4/FIR Interpolation  FilterSource=Dialog parameters  h=[6 0 -19 0 47 0 -100 0 192 0 -342 0 572 0 -914 0 1409 0 -2119 0 3152 0 -4729 0 7420 0 -13334 0 41527 65536 41527 0 -13334 0 7420 0 -4729 0 3152 0 -2119 0 1409 0 -914 0 572 0 -342 0 192 0 -100 0 47 0 -19 0 6 ]*2^-16  L=2  FilterObject=FINTERP  framing=Enforce single-rate processing  outputBufInitCond=0  roundingMode=Round  overflowMode=on  firstCoeffMode=Binary point scaling  firstCoeffWordLength=18  firstCoeffFracLength=16  firstCoeffDataTypeStr=fixdt(1,18,16)  firstCoeffMin=[]  firstCoeffMax=[]  firstCoeffLastDataTypeStr=fixdt(1,18,16)  outputMode=Binary point scaling  outputWordLength=18  outputFracLength=17  outputDataTypeStr=fixdt(1,18,17)  outputMin=[]  outputMax=[]  outputLastDataTypeStr=fixdt(1,18,17)
  fir2 : dspmlti4/FIR Interpolation  FilterSource=Dialog parameters  h=[-12 0 84 0 -336 0 1006 0 -2691 0 10141 16384 10141 0 -2691 0 1006 0 -336 0 84 0 -12 ]*2^-14  L=2  FilterObject=FINTERP  framing=Enforce single-rate processing  outputBufInitCond=0  roundingMode=Round  overflowMode=on  firstCoeffMode=Binary point scaling  firstCoeffWordLength=16  firstCoeffFracLength=14  firstCoeffDataTypeStr=fixdt(1,16,14)  firstCoeffMin=[]  firstCoeffMax=[]  firstCoeffLastDataTypeStr=fixdt(1,16,14)  outputMode=Binary point scaling  outputWordLength=18  outputFracLength=17  outputDataTypeStr=fixdt(1,18,17)  outputMin=[]  outputMax=[]  outputLastDataTypeStr=fixdt(1,18,17)
  fir3 : dspmlti4/FIR Interpolation  FilterSource=Dialog parameters  h=[29 0 -214 0 1209 2048 1209 0 -214 0 29 ]*2^-11  L=2  FilterObject=FINTERP  framing=Enforce single-rate processing  outputBufInitCond=0  roundingMode=Round  overflowMode=on  firstCoeffMode=Binary point scaling  firstCoeffWordLength=13  firstCoeffFracLength=11  firstCoeffDataTypeStr=fixdt(1,13,11)  firstCoeffMin=[]  firstCoeffMax=[]  firstCoeffLastDataTypeStr=fixdt(1,13,11)  outputMode=Binary point scaling  outputWordLength=17  outputFracLength=16  outputDataTypeStr=fixdt(1,17,16)  outputMin=[]  outputMax=[]  outputLastDataTypeStr=fixdt(1,17,16)
  fir4 : dspmlti4/FIR Interpolation  FilterSource=Dialog parameters  h=[3 0 -25 0 150 256 150 0 -25 0 3 ]*2^-8  L=2  FilterObject=FINTERP  framing=Enforce single-rate processing  outputBufInitCond=0  roundingMode=Round  overflowMode=on  firstCoeffMode=Binary point scaling  firstCoeffWordLength=10  firstCoeffFracLength=8  firstCoeffDataTypeStr=fixdt(1,10,8)  firstCoeffMin=[]  firstCoeffMax=[]  firstCoeffLastDataTypeStr=fixdt(1,10,8)  outputMode=Binary point scaling  outputWordLength=17  outputFracLength=16  outputDataTypeStr=fixdt(1,17,16)  outputMin=[]  outputMax=[]  outputLastDataTypeStr=fixdt(1,17,16)
  fir4_5 : dspmlti4/FIR Interpolation  FilterSource=Dialog parameters  h=[3 0 -25 0 150 256 150 0 -25 0 3 ]*2^-8  L=2  FilterObject=FINTERP  framing=Enforce single-rate processing  outputBufInitCond=0  roundingMode=Round  overflowMode=on  firstCoeffMode=Binary point scaling  firstCoeffWordLength=10  firstCoeffFracLength=8  firstCoeffDataTypeStr=fixdt(1,10,8)  firstCoeffMin=[]  firstCoeffMax=[]  firstCoeffLastDataTypeStr=fixdt(1,10,8)  outputMode=Binary point scaling  outputWordLength=17  outputFracLength=16  outputDataTypeStr=fixdt(1,17,16)  outputMin=[]  outputMax=[]  outputLastDataTypeStr=fixdt(1,17,16)
  fir4_6 : dspmlti4/FIR Interpolation  FilterSource=Dialog parameters  h=[3 0 -25 0 150 256 150 0 -25 0 3 ]*2^-8  L=2  FilterObject=FINTERP  framing=Enforce single-rate processing  outputBufInitCond=0  roundingMode=Round  overflowMode=on  firstCoeffMode=Binary point scaling  firstCoeffWordLength=10  firstCoeffFracLength=8  firstCoeffDataTypeStr=fixdt(1,10,8)  firstCoeffMin=[]  firstCoeffMax=[]  firstCoeffLastDataTypeStr=fixdt(1,10,8)  outputMode=Binary point scaling  outputWordLength=17  outputFracLength=16  outputDataTypeStr=fixdt(1,17,16)  outputMin=[]  outputMax=[]  outputLastDataTypeStr=fixdt(1,17,16)
  fir5_7 : dspmlti4/FIR Interpolation  FilterSource=Dialog parameters  h=[-1 0 9 16 9 0 -1]*2^-4  L=2  FilterObject=FINTERP  framing=Enforce single-rate processing  outputBufInitCond=0  roundingMode=Round  overflowMode=on  firstCoeffMode=Binary point scaling  firstCoeffWordLength=6  firstCoeffFracLength=4  firstCoeffDataTypeStr=fixdt(1,6,4)  firstCoeffMin=[]  firstCoeffMax=[]  firstCoeffLastDataTypeStr=fixdt(1,6,4)  outputMode=Binary point scaling  outputWordLength=16  outputFracLength=15  outputDataTypeStr=fixdt(1,16,15)  outputMin=[]  outputMax=[]  outputLastDataTypeStr=fixdt(1,16,15)
  fir5_8 : dspmlti4/FIR Interpolation  FilterSource=Dialog parameters  h=[-1 0 9 16 9 0 -1]*2^-4  L=2  FilterObject=FINTERP  framing=Enforce single-rate processing  outputBufInitCond=0  roundingMode=Round  overflowMode=on  firstCoeffMode=Binary point scaling  firstCoeffWordLength=6  firstCoeffFracLength=4  firstCoeffDataTypeStr=fixdt(1,6,4)  firstCoeffMin=[]  firstCoeffMax=[]  firstCoeffLastDataTypeStr=fixdt(1,6,4)  outputMode=Binary point scaling  outputWordLength=16  outputFracLength=15  outputDataTypeStr=fixdt(1,16,15)  outputMin=[]  outputMax=[]  outputLastDataTypeStr=fixdt(1,16,15)
  " Out1" : Outport  VectorParamsAs1DForOutWhenUnconnected=off
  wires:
  fir4_5/1 -> fir4_6/1
  fir5_7/1 -> fir5_8/1
  "In1 "/1 -> fir1/1
  fir1/1 -> fir2/1
  fir2/1 -> fir3/1
  fir3/1 -> fir4/1
  fir4/1 -> fir4_5/1
  fir5_8/1 -> " Out1"/1
  fir4_6/1 -> fir5_7/1

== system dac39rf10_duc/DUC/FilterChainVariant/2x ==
  In1 : Inport
  fir1 : dspmlti4/FIR Interpolation  FilterSource=Dialog parameters  h=[6 0 -19 0 47 0 -100 0 192 0 -342 0 572 0 -914 0 1409 0 -2119 0 3152 0 -4729 0 7420 0 -13334 0 41527 65536 41527 0 -13334 0 7420 0 -4729 0 3152 0 -2119 0 1409 0 -914 0 572 0 -342 0 192 0 -100 0 47 0 -19 0 6 ]*2^-16  L=2  FilterObject=FINTERP  framing=Enforce single-rate processing  outputBufInitCond=0  roundingMode=Round  overflowMode=on  firstCoeffMode=Binary point scaling  firstCoeffWordLength=18  firstCoeffFracLength=16  firstCoeffDataTypeStr=fixdt(1,18,16)  firstCoeffMin=[]  firstCoeffMax=[]  firstCoeffLastDataTypeStr=fixdt(1,18,16)  outputMode=Binary point scaling  outputWordLength=16  outputFracLength=15  outputDataTypeStr=fixdt(1,16,15)  outputMin=[]  outputMax=[]  outputLastDataTypeStr=fixdt(1,16,15)
  Out1 : Outport  VectorParamsAs1DForOutWhenUnconnected=off
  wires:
  In1/1 -> fir1/1
  fir1/1 -> Out1/1

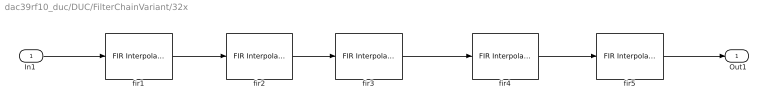
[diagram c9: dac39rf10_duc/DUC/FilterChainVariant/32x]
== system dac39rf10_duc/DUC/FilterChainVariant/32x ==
  "In1 " : Inport
  fir1 : dspmlti4/FIR Interpolation  FilterSource=Dialog parameters  h=[6 0 -19 0 47 0 -100 0 192 0 -342 0 572 0 -914 0 1409 0 -2119 0 3152 0 -4729 0 7420 0 -13334 0 41527 65536 41527 0 -13334 0 7420 0 -4729 0 3152 0 -2119 0 1409 0 -914 0 572 0 -342 0 192 0 -100 0 47 0 -19 0 6 ]*2^-16  L=2  FilterObject=FINTERP  framing=Enforce single-rate processing  outputBufInitCond=0  roundingMode=Round  overflowMode=on  firstCoeffMode=Binary point scaling  firstCoeffWordLength=18  firstCoeffFracLength=16  firstCoeffDataTypeStr=fixdt(1,18,16)  firstCoeffMin=[]  firstCoeffMax=[]  firstCoeffLastDataTypeStr=fixdt(1,18,16)  outputMode=Binary point scaling  outputWordLength=18  outputFracLength=17  outputDataTypeStr=fixdt(1,18,17)  outputMin=[]  outputMax=[]  outputLastDataTypeStr=fixdt(1,18,17)
  fir2 : dspmlti4/FIR Interpolation  FilterSource=Dialog parameters  h=[-12 0 84 0 -336 0 1006 0 -2691 0 10141 16384 10141 0 -2691 0 1006 0 -336 0 84 0 -12 ]*2^-14  L=2  FilterObject=FINTERP  framing=Enforce single-rate processing  outputBufInitCond=0  roundingMode=Round  overflowMode=on  firstCoeffMode=Binary point scaling  firstCoeffWordLength=16  firstCoeffFracLength=14  firstCoeffDataTypeStr=fixdt(1,16,14)  firstCoeffMin=[]  firstCoeffMax=[]  firstCoeffLastDataTypeStr=fixdt(1,16,14)  outputMode=Binary point scaling  outputWordLength=18  outputFracLength=17  outputDataTypeStr=fixdt(1,18,17)  outputMin=[]  outputMax=[]  outputLastDataTypeStr=fixdt(1,18,17)
  fir3 : dspmlti4/FIR Interpolation  FilterSource=Dialog parameters  h=[29 0 -214 0 1209 2048 1209 0 -214 0 29 ]*2^-11  L=2  FilterObject=FINTERP  framing=Enforce single-rate processing  outputBufInitCond=0  roundingMode=Round  overflowMode=on  firstCoeffMode=Binary point scaling  firstCoeffWordLength=13  firstCoeffFracLength=11  firstCoeffDataTypeStr=fixdt(1,13,11)  firstCoeffMin=[]  firstCoeffMax=[]  firstCoeffLastDataTypeStr=fixdt(1,13,11)  outputMode=Binary point scaling  outputWordLength=17  outputFracLength=16  outputDataTypeStr=fixdt(1,17,16)  outputMin=[]  outputMax=[]  outputLastDataTypeStr=fixdt(1,17,16)
  fir4 : dspmlti4/FIR Interpolation  FilterSource=Dialog parameters  h=[3 0 -25 0 150 256 150 0 -25 0 3 ]*2^-8  L=2  FilterObject=FINTERP  framing=Enforce single-rate processing  outputBufInitCond=0  roundingMode=Round  overflowMode=on  firstCoeffMode=Binary point scaling  firstCoeffWordLength=10  firstCoeffFracLength=8  firstCoeffDataTypeStr=fixdt(1,10,8)  firstCoeffMin=[]  firstCoeffMax=[]  firstCoeffLastDataTypeStr=fixdt(1,10,8)  outputMode=Binary point scaling  outputWordLength=17  outputFracLength=16  outputDataTypeStr=fixdt(1,17,16)  outputMin=[]  outputMax=[]  outputLastDataTypeStr=fixdt(1,17,16)
  fir5 : dspmlti4/FIR Interpolation  FilterSource=Dialog parameters  h=[-1 0 9 16 9 0 -1]*2^-4  L=2  FilterObject=FINTERP  framing=Enforce single-rate processing  outputBufInitCond=0  roundingMode=Round  overflowMode=on  firstCoeffMode=Binary point scaling  firstCoeffWordLength=6  firstCoeffFracLength=4  firstCoeffDataTypeStr=fixdt(1,6,4)  firstCoeffMin=[]  firstCoeffMax=[]  firstCoeffLastDataTypeStr=fixdt(1,6,4)  outputMode=Binary point scaling  outputWordLength=16  outputFracLength=15  outputDataTypeStr=fixdt(1,16,15)  outputMin=[]  outputMax=[]  outputLastDataTypeStr=fixdt(1,16,15)
  " Out1" : Outport  VectorParamsAs1DForOutWhenUnconnected=off
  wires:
  fir4/1 -> fir5/1
  fir3/1 -> fir4/1
  fir2/1 -> fir3/1
  fir1/1 -> fir2/1
  "In1 "/1 -> fir1/1
  fir5/1 -> " Out1"/1

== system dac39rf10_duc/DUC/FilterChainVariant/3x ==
  In1 : Inport
  fir3x : dspmlti4/FIR Interpolation  FilterSource=Dialog parameters  h=[-38 -38 0 83 117 0 -214 -281 0 464 584 0 -900 -1102 0 1612 1929 0 -2713 -3190 0 4346 5040 0 -6699 -7684 0 10023 11408 0 -14701 -16661 0 21389 24260 0 -31417 -35960 0 48101 56540 0 -82781 -105224 0 215190 432780 524288 432780 215190 0 -105224 -82781 0 56540 48101 0 -35960 -31417 0 24260 21389 0 -16661 -14701 0 11408 10023 0 -7684 -6699 0 5040 4346 0 -3190 -2713 0 1929 1612 0 -1102 -900 0 584 464 0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  L=3  FilterObject=FINTERP  framing=Enforce single-rate processing  outputBufInitCond=0  roundingMode=Round  overflowMode=on  firstCoeffMode=Binary point scaling  firstCoeffWordLength=21  firstCoeffFracLength=19  firstCoeffDataTypeStr=fixdt(1,21,19)  firstCoeffMin=[]  firstCoeffMax=[]  firstCoeffLastDataTypeStr=fixdt(1,21,19)  outputMode=Binary point scaling  outputWordLength=16  outputFracLength=15  outputDataTypeStr=fixdt(1,16,15)  outputMin=[]  outputMax=[]  outputLastDataTypeStr=fixdt(1,16,15)
  Out1 : Outport  VectorParamsAs1DForOutWhenUnconnected=off
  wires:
  fir3x/1 -> Out1/1
  In1/1 -> fir3x/1

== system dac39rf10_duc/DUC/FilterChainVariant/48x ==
  "In1 " : Inport
  fir2 : dspmlti4/FIR Interpolation  FilterSource=Dialog parameters  h=[-12 0 84 0 -336 0 1006 0 -2691 0 10141 16384 10141 0 -2691 0 1006 0 -336 0 84 0 -12 ]*2^-14  L=2  FilterObject=FINTERP  framing=Enforce single-rate processing  outputBufInitCond=0  roundingMode=Round  overflowMode=on  firstCoeffMode=Binary point scaling  firstCoeffWordLength=16  firstCoeffFracLength=14  firstCoeffDataTypeStr=fixdt(1,16,14)  firstCoeffMin=[]  firstCoeffMax=[]  firstCoeffLastDataTypeStr=fixdt(1,16,14)  outputMode=Binary point scaling  outputWordLength=18  outputFracLength=17  outputDataTypeStr=fixdt(1,18,17)  outputMin=[]  outputMax=[]  outputLastDataTypeStr=fixdt(1,18,17)
  fir3 : dspmlti4/FIR Interpolation  FilterSource=Dialog parameters  h=[29 0 -214 0 1209 2048 1209 0 -214 0 29 ]*2^-11  L=2  FilterObject=FINTERP  framing=Enforce single-rate processing  outputBufInitCond=0  roundingMode=Round  overflowMode=on  firstCoeffMode=Binary point scaling  firstCoeffWordLength=13  firstCoeffFracLength=11  firstCoeffDataTypeStr=fixdt(1,13,11)  firstCoeffMin=[]  firstCoeffMax=[]  firstCoeffLastDataTypeStr=fixdt(1,13,11)  outputMode=Binary point scaling  outputWordLength=17  outputFracLength=16  outputDataTypeStr=fixdt(1,17,16)  outputMin=[]  outputMax=[]  outputLastDataTypeStr=fixdt(1,17,16)
  fir3x : dspmlti4/FIR Interpolation  FilterSource=Dialog parameters  h=[-38 -38 0 83 117 0 -214 -281 0 464 584 0 -900 -1102 0 1612 1929 0 -2713 -3190 0 4346 5040 0 -6699 -7684 0 10023 11408 0 -14701 -16661 0 21389 24260 0 -31417 -35960 0 48101 56540 0 -82781 -105224 0 215190 432780 524288 432780 215190 0 -105224 -82781 0 56540 48101 0 -35960 -31417 0 24260 21389 0 -16661 -14701 0 11408 10023 0 -7684 -6699 0 5040 4346 0 -3190 -2713 0 1929 1612 0 -1102 -900 0 584 464 0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  L=3  FilterObject=FINTERP  framing=Enforce single-rate processing  outputBufInitCond=0  roundingMode=Round  overflowMode=on  firstCoeffMode=Binary point scaling  firstCoeffWordLength=21  firstCoeffFracLength=19  firstCoeffDataTypeStr=fixdt(1,21,19)  firstCoeffMin=[]  firstCoeffMax=[]  firstCoeffLastDataTypeStr=fixdt(1,21,19)  outputMode=Binary point scaling  outputWordLength=18  outputFracLength=17  outputDataTypeStr=fixdt(1,18,17)  outputMin=[]  outputMax=[]  outputLastDataTypeStr=fixdt(1,18,17)
  fir4 : dspmlti4/FIR Interpolation  FilterSource=Dialog parameters  h=[3 0 -25 0 150 256 150 0 -25 0 3 ]*2^-8  L=2  FilterObject=FINTERP  framing=Enforce single-rate processing  outputBufInitCond=0  roundingMode=Round  overflowMode=on  firstCoeffMode=Binary point scaling  firstCoeffWordLength=10  firstCoeffFracLength=8  firstCoeffDataTypeStr=fixdt(1,10,8)  firstCoeffMin=[]  firstCoeffMax=[]  firstCoeffLastDataTypeStr=fixdt(1,10,8)  outputMode=Binary point scaling  outputWordLength=17  outputFracLength=16  outputDataTypeStr=fixdt(1,17,16)  outputMin=[]  outputMax=[]  outputLastDataTypeStr=fixdt(1,17,16)
  fir5 : dspmlti4/FIR Interpolation  FilterSource=Dialog parameters  h=[-1 0 9 16 9 0 -1]*2^-4  L=2  FilterObject=FINTERP  framing=Enforce single-rate processing  outputBufInitCond=0  roundingMode=Round  overflowMode=on  firstCoeffMode=Binary point scaling  firstCoeffWordLength=6  firstCoeffFracLength=4  firstCoeffDataTypeStr=fixdt(1,6,4)  firstCoeffMin=[]  firstCoeffMax=[]  firstCoeffLastDataTypeStr=fixdt(1,6,4)  outputMode=Binary point scaling  outputWordLength=16  outputFracLength=15  outputDataTypeStr=fixdt(1,16,15)  outputMin=[]  outputMax=[]  outputLastDataTypeStr=fixdt(1,16,15)
  " Out1" : Outport  VectorParamsAs1DForOutWhenUnconnected=off
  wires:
  fir5/1 -> " Out1"/1
  "In1 "/1 -> fir3x/1
  fir3x/1 -> fir2/1
  fir2/1 -> fir3/1
  fir3/1 -> fir4/1
  fir4/1 -> fir5/1

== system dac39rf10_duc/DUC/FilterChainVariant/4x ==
  "In1 " : Inport
  fir1 : dspmlti4/FIR Interpolation  FilterSource=Dialog parameters  h=[6 0 -19 0 47 0 -100 0 192 0 -342 0 572 0 -914 0 1409 0 -2119 0 3152 0 -4729 0 7420 0 -13334 0 41527 65536 41527 0 -13334 0 7420 0 -4729 0 3152 0 -2119 0 1409 0 -914 0 572 0 -342 0 192 0 -100 0 47 0 -19 0 6 ]*2^-16  L=2  FilterObject=FINTERP  framing=Enforce single-rate processing  outputBufInitCond=0  roundingMode=Round  overflowMode=on  firstCoeffMode=Binary point scaling  firstCoeffWordLength=18  firstCoeffFracLength=16  firstCoeffDataTypeStr=fixdt(1,18,16)  firstCoeffMin=[]  firstCoeffMax=[]  firstCoeffLastDataTypeStr=fixdt(1,18,16)  outputMode=Binary point scaling  outputWordLength=18  outputFracLength=17  outputDataTypeStr=fixdt(1,18,17)  outputMin=[]  outputMax=[]  outputLastDataTypeStr=fixdt(1,18,17)
  fir2 : dspmlti4/FIR Interpolation  FilterSource=Dialog parameters  h=[-12 0 84 0 -336 0 1006 0 -2691 0 10141 16384 10141 0 -2691 0 1006 0 -336 0 84 0 -12 ]*2^-14  L=2  FilterObject=FINTERP  framing=Enforce single-rate processing  outputBufInitCond=0  roundingMode=Round  overflowMode=on  firstCoeffMode=Binary point scaling  firstCoeffWordLength=16  firstCoeffFracLength=14  firstCoeffDataTypeStr=fixdt(1,16,14)  firstCoeffMin=[]  firstCoeffMax=[]  firstCoeffLastDataTypeStr=fixdt(1,16,14)  outputMode=Binary point scaling  outputWordLength=16  outputFracLength=15  outputDataTypeStr=fixdt(1,16,15)  outputMin=[]  outputMax=[]  outputLastDataTypeStr=fixdt(1,16,15)
  " Out1" : Outport  VectorParamsAs1DForOutWhenUnconnected=off
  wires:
  "In1 "/1 -> fir1/1
  fir1/1 -> fir2/1
  fir2/1 -> " Out1"/1
